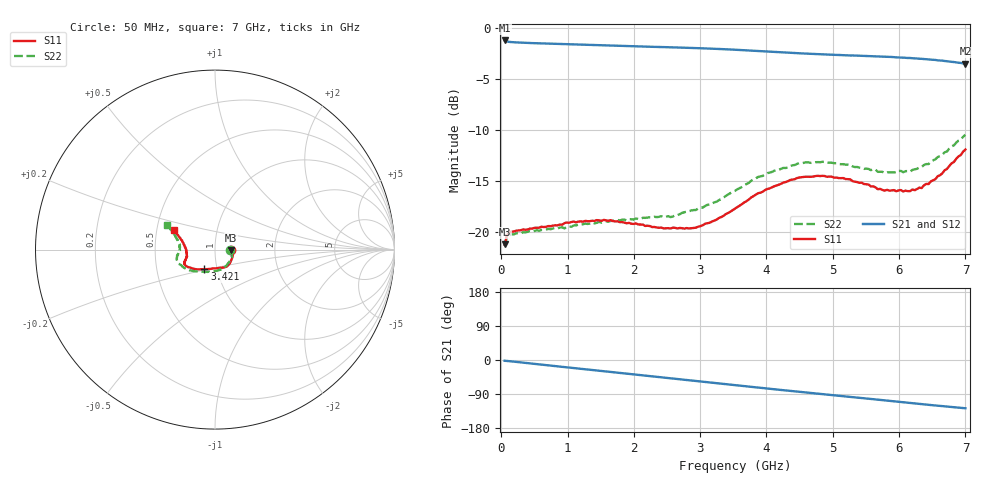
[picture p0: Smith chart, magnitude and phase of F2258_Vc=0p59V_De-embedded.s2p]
! Integrated Device Technology
! Corporate Headquarters
! 6024 Silver Creek Valley Road
! San Jose, CA 95138  USA
! Phone:  1-408-284-8200
! Toll Free:  1-800-223-1366
! Webpage:  http://www.idt.com/
! Timing and RF Division
! 515 Groton Road, Suite 102
! Westford, MA 01886-6024
! Device:  F2258
! Description: Voltage Variable RF Attenuator
! Frequency:  50.0 -  6000.00 MHz
! Package:  3x3 mm Thin QFN Plastic Package: 16 pin
! Ports:  2 RF, 2 DC
!  Pin  1  = NC
!  Pin  2  = NC
!  Pin  3  = RF2  = Port 2
!  Pin  4  = GND
!  Pin  5  = Vdd
!  Pin  6  = NC
!  Pin  7  = VCTRL
!  Pin  8  = NC
!  Pin  9  = GND
!  Pin 10  = RF1  = Port 1
!  Pin 11  = NC
!  Pin 12  = NC
!  Pin 13  = NC
!  Pin 14  = NC
!  Pin 15  = NC
!  Pin 16  = NC
! Vcntrl:  0.590 Volts
! Vdd:  +3.300 Volts
! Current:  1.107 mA
! Data:  The device was measured on a the F2258 evaluation board which has
!  individual transmission lines to the RF pins.  Data was collected
!  using a calibrated network analyzer.  The evaluation board was
!  de-embedded using a TRL calibration technique.
!  The reference plane is the edge of the package pin.
! Misc:  SN 10
!  Action Tracker AT0285
! Date Measured:  2014-12-10
! Date:  2016-01-13  MJV
! Note:
!  Integrated Device Technology supplies this data as a sample of measured
!  data at the package pin for this product.  Your particular data for this
!  product may vary.
!  Data was taken at 25 degrees C.
!  Integrated Device Technology reserves the right to change this data at anytime.
!Freq_(GHz)  S11M_(dB)  S11P_(deg)  S21M_(dB)  S21P_(deg)  S12M_(dB)  S12P_(deg)  S22M_(dB)  S22P_(deg)
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# GHz S dB R 50
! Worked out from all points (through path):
!   201 points, 50 MHz to 7 GHz, reference 50 ohm
!   highest |S21| = -1.25 dB at 50 MHz (marker M1); lowest = -3.5 dB at 7 GHz (marker M2)
!   group delay of S21, straight-line fit = 50.5 ps
!   lowest |S11| = -21.2 dB at 50 MHz (marker M3), VSWR 1.19, Z = 59.5 - j0.484 ohm
!   |S11| at or under -10 dB: start of sweep to end of sweep
!   |S22| runs from -21.4 to -10.5 dB; largest |S21 - S12| = 0.00056
!   S11 on the Smith chart (normalised r, x): 50 MHz: 1.19, -0.01; 3.421 GHz: 0.87, -0.19; 7 GHz: 0.62, +0.14
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0.05  -21.20 -2.7  -1.25 -2.0  -1.25 -2.0  -21.37 -2.9
0.08475  -20.33 -4.3  -1.35 -2.5  -1.35 -2.5  -20.53 -4.6
0.15425  -19.94 -6.8  -1.41 -3.7  -1.41 -3.7  -20.21 -7.9
0.71025  -19.40 -28.3  -1.55 -14.1  -1.55 -14.2  -19.68 -33.0
1.2315  -18.98 -46.8  -1.67 -23.9  -1.66 -23.9  -19.23 -55.6
1.6485  -18.83 -57.0  -1.76 -31.5  -1.75 -31.5  -18.91 -68.6
2.37825  -19.58 -74.7  -1.89 -44.8  -1.89 -44.8  -18.51 -87.7
2.552  -19.64 -80.1  -1.92 -48.0  -1.91 -48.0  -18.53 -93.0
2.93425  -19.56 -95.9  -2.00 -55.1  -1.99 -55.1  -17.84 -106.7
3.247  -18.78 -109.9  -2.07 -61.0  -2.07 -61.0  -17.02 -119.1
3.42075  -18.12 -118.5  -2.12 -64.3  -2.12 -64.3  -16.31 -126.3
3.525  -17.72 -122.5  -2.15 -66.3  -2.16 -66.2  -15.96 -130.2
4.0115  -15.79 -139.6  -2.33 -75.3  -2.33 -75.3  -14.23 -146.6
4.46325  -14.70 -149.4  -2.49 -83.5  -2.50 -83.4  -13.32 -158.3
4.7065  -14.57 -152.8  -2.57 -87.7  -2.57 -87.7  -13.21 -162.7
5.2625  -14.83 -159.2  -2.72 -97.4  -2.73 -97.4  -13.40 -171.3
5.6795  -15.80 -164.9  -2.81 -104.6  -2.81 -104.6  -14.10 -177.2
5.85325  -15.93 -169.0  -2.86 -107.7  -2.86 -107.7  -14.15 178.1
6.166  -15.99 -177.2  -2.96 -113.3  -2.97 -113.3  -14.09 171.8
6.33975  -15.69 175.7  -3.05 -116.4  -3.05 -116.4  -13.62 167.2
6.6525  -14.24 164.2  -3.22 -121.9  -3.23 -121.9  -12.41 160.3
7  -11.92 154.3  -3.52 -127.4  -3.53 -127.4  -10.47 152.7
